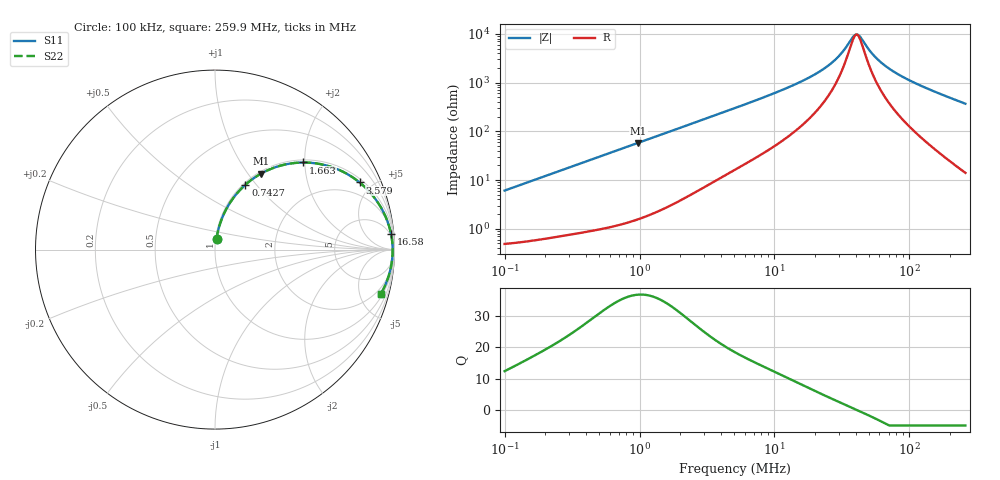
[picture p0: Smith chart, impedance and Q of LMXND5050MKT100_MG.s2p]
! LMXND5050MKT100_MG  S-PARAMETER MODEL  ( General Type )
! Model Generated by TAIYO YUDEN Corporation (http://www.ty-top.com)
! Version 1.0
! TAIYO YUDEN Control No. 191023NI43SB-FBB
! Copyright(c) 2019 TAIYO YUDEN CO.,LTD. All Rights Reserved.
! Product Description (link to TY-COMPAS)
! https://ds.yuden.co.jp/TYCOMPAS/or/detail?pn=LMXND5050MKT100MMG&u=M
! Products Name : Inductors
! Characteristics :
!  Inductance : 10 uH , SRF(min) : 26 MHz , DC Resistance(max) : 0.504 Ohm
!  Rated Current : Saturation :1400 mA , Temp Rise : 850 mA
!  Case Size : 4.9 x 4.9 / 0.193 x 0.193 [mm/inch] , Thickness : 1.2 / 0.047 [mm/inch]
!  (Conditions: Temperature = 25 degC , DC Bias Current/Voltage = 0A / 0V)
! External Node Assignments :
!  1  o---GGG---o  2
! GND o---------o GND
! Frequency Range : 0.1MHz  -  259.929867MHz  [ 402 STEP ]
# MHz S RI R 50
! Freq[MHz].  S11 Real  S11 Imag  S21 Real  S21 Imag  S12 Real  S12 Imag  S22 Real  S22 Imag
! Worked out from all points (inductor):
!   401 points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, 100 kHz to 259.9 MHz, reference 50 ohm
!   read as one part in series: L = 9.64 uH near 104 kHz
!   highest Q = 36.9 at 977.9 kHz (marker M1), where L = 9.43 uH
!   self-resonance near 40.16 MHz
!   S11 on the Smith chart (normalised r, x): 100 kHz: 1.01, +0.12; 742.7 kHz: 1.02, +0.88; 1.663 MHz: 1.06, +1.97; 3.579 MHz: 1.19, +4.21; 16.58 MHz: 4, +22; 259.9 MHz: 1.28, -7.37
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0.1  0.00849 0.0599  0.9915 -0.0599  0.9915 -0.0599  0.00849 0.0599
0.37324  0.0544 0.209  0.9456 -0.209  0.9456 -0.209  0.0544 0.209
0.742657  0.1696 0.3614  0.8304 -0.3614  0.8304 -0.3614  0.1696 0.3614
0.977931  0.2571 0.4237  0.7429 -0.4237  0.7429 -0.4237  0.2571 0.4237
1.393082  0.4072 0.4774  0.5928 -0.4774  0.5928 -0.4774  0.4072 0.4774
1.662689  0.4917 0.4853  0.5083 -0.4853  0.5083 -0.4853  0.4917 0.4853
2.322429  0.6479 0.4606  0.3521 -0.4606  0.3521 -0.4606  0.6479 0.4606
3.578982  0.806 0.3739  0.194 -0.3739  0.194 -0.3739  0.806 0.3739
5.098332  0.8879 0.2896  0.1121 -0.2896  0.1121 -0.2896  0.8879 0.2896
9.946971  0.9614 0.1562  0.0386 -0.1562  0.0386 -0.1562  0.9614 0.1562
16.58275  0.9812 0.0854  0.0188 -0.0854  0.0188 -0.0854  0.9812 0.0854
19.02902  0.984 0.07  0.016 -0.07  0.016 -0.07  0.984 0.07
23.62246  0.987 0.048  0.013 -0.048  0.013 -0.048  0.987 0.048
28.19417  0.9886 0.0316  0.0114 -0.0316  0.0114 -0.0316  0.9886 0.0316
32.35335  0.9893 0.0194  0.0107 -0.0194  0.0107 -0.0194  0.9893 0.0194
37.86312  0.9898 0.00593  0.0102 -0.00593  0.0102 -0.00593  0.9898 0.00593
40.16316  0.9898 0.000919  0.0102 -0.000919  0.0102 -0.000919  0.9898 0.000919
43.44866  0.9898 -0.00576  0.0102 0.00576  0.0102 0.00576  0.9898 -0.00576
56.09953  0.9892 -0.0279  0.0108 0.0279  0.0108 0.0279  0.9892 -0.0279
71.02397  0.9875 -0.0499  0.0125 0.0499  0.0125 0.0499  0.9875 -0.0499
118.4051  0.9781 -0.108  0.0219 0.108  0.0219 0.108  0.9781 -0.108
259.9299  0.9234 -0.2475  0.0766 0.2475  0.0766 0.2475  0.9234 -0.2475
